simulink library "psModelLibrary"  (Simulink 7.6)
settings: Solver=ode45  SolverMode=SingleTasking  StartTime=0.0  StopTime=10.0  RelTol=1e-3
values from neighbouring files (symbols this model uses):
  psSimStruct = []    [psStartUp.m]
undefined symbols (not defined in the file or in its folder): psValve, psVolume, Restriction

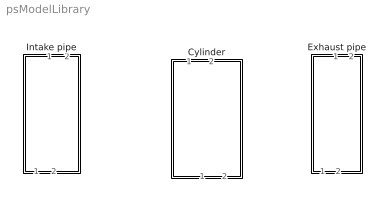
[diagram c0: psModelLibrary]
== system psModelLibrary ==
  Cylinder : Subsystem  mask{thetaOffset=0, CylNbr=1}
      mask prompts: thetaOffset "thetaOffset [rad]"; CylNbr "Cylinder Number"
  Exhaust pipe : Subsystem  mask{CylNbr=1}
      mask prompts: CylNbr "Cylinder Number"
  Intake pipe : Subsystem  mask{CylNbr=1}
      mask prompts: CylNbr "Cylinder Number"

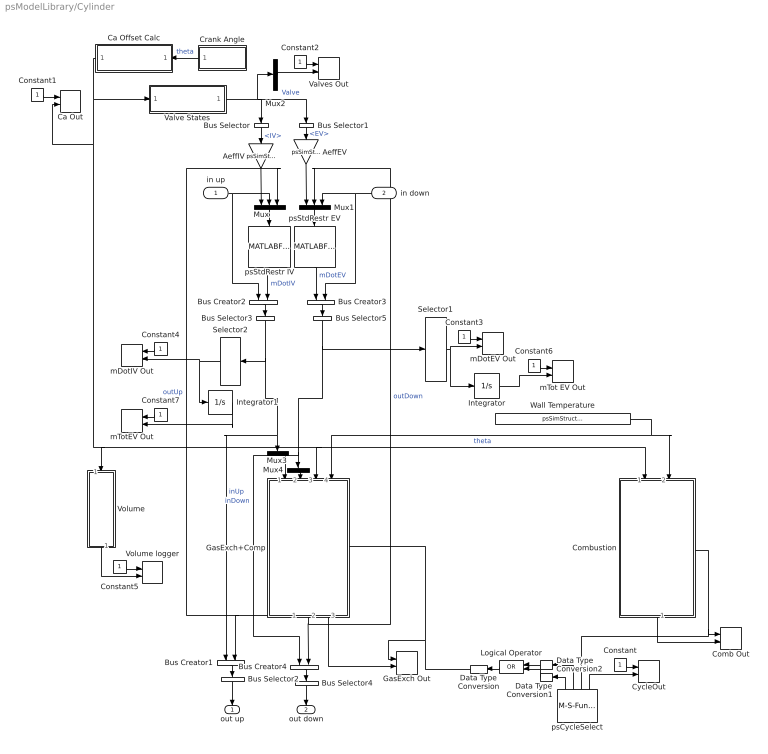
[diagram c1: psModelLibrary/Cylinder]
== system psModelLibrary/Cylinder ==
  in up : Inport
  in down : Inport  Port=2
  AeffEV : Gain  Gain=psSimStruct.psGeometry.Ath_EV*psSimStruct.psGeometry.Cd_EV
  AeffIV : Gain  Gain=psSimStruct.psGeometry.Ath_IV*psSimStruct.psGeometry.Cd_IV
  Bus Creator{1..4} (4 alike) : BusCreator  Inputs=2
  Bus Selector : BusSelector  OutputSignals=IV
  Bus Selector1 : BusSelector  OutputSignals=EV
  Bus Selector2 : BusSelector  OutputSignals=inUp.mDotIV,outUp.state  OutputAsBus=on
  Bus Selector3 : BusSelector  OutputSignals=mDotIV,signal1.state  OutputAsBus=on
  Bus Selector4 : BusSelector  OutputSignals=inDown.mDotEV,outDown.state  OutputAsBus=on
  Bus Selector5 : BusSelector  OutputSignals=mDotEV,signal2.state  OutputAsBus=on
  Ca Offset Calc : Subsystem
  Ca Out : M-S-Function  FunctionName=psToWorkspace  Parameters=1,int16('theta'),CylNbr
  Comb Out : M-S-Function  FunctionName=psToWorkspace  Parameters=9+2*psSimStruct.psThermProp.K,int16('pcb Vb Tb Vu Tu'),CylNbr
  Combustion : Subsystem  TreatAsAtomicUnit=on
  Constant{,1..7} (8 alike) : Constant
  Crank Angle : Subsystem
  CycleOut : M-S-Function  FunctionName=psToWorkspace  Parameters=1,int16('phase'),CylNbr
  Data Type Conversion : DataTypeConversion
  Data Type Conversion1 : DataTypeConversion
  Data Type Conversion2 : DataTypeConversion
  GasExch Out : M-S-Function  FunctionName=psToWorkspace  Parameters=psSimStruct.psThermProp.K+4,int16('pge Vge Tge'),CylNbr
  GasExch+Comp : Subsystem  Priority=1
  Integrator : Integrator
  Integrator1 : Integrator
  Logical Operator : Logic  Operator=OR  AllPortsSameDT=off  OutDataTypeStr=boolean
  Mux : Mux  Inputs=3
  Mux1 : Mux  Inputs=3
  Mux2 : Mux  Inputs=1
  Mux3 : Mux  Inputs=1
  Mux4 : Mux  Inputs=1
  Selector1 : Selector  IndexOptions=Index vector (dialog)  Indices=[1]  OutputSizes=[(-2)]
  Selector2 : Selector  IndexOptions=Index vector (dialog)  Indices=[1]  OutputSizes=[(-2)]
  Valve States : Subsystem
  Valves Out : M-S-Function  FunctionName=psToWorkspace  Parameters=2,int16('uIV uEV'),CylNbr
  Volume : Subsystem
  Volume logger : M-S-Function  FunctionName=psToWorkspace  Parameters=1,int16('V'),CylNbr
  Wall Temperature : Constant  Value=psSimStruct.psModel.T_Wall
  mDotEV Out : M-S-Function  FunctionName=psToWorkspace  Parameters=1,int16('mDotEV'),CylNbr
  mDotIV Out : M-S-Function  FunctionName=psToWorkspace  Parameters=1,int16('mDotIV'),CylNbr
  mTot EV Out : M-S-Function  FunctionName=psToWorkspace  Parameters=1,int16('mTotEV'),CylNbr
  mTotEV Out : M-S-Function  FunctionName=psToWorkspace  Parameters=1,int16('mTotIV'),CylNbr
  psCycleSelect : M-S-Function  FunctionName=psCycleSelect  Parameters=caOffset  mask{caOffset=thetaOffset}
      mask prompts: caOffset "caOffset [rad]"
  psStdRestr EV : MATLABFcn  MATLABFcn=psStdRestr  OutputDimensions=1  OutputSignalType=real
  psStdRestr IV : MATLABFcn  MATLABFcn=psStdRestr  OutputDimensions=1  OutputSignalType=real
  out up : Outport
  out down : Outport  Port=2
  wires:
  Constant7/1 -> mTotEV Out/1
  Integrator1/1 -> mTotEV Out/2
  Constant6/1 -> mTot EV Out/1
  Integrator/1 -> mTot EV Out/2
  Data Type Conversion2/1 -> Logical Operator/1
  Data Type Conversion1/1 -> Logical Operator/2
  Data Type Conversion/1 -> GasExch Out/1, GasExch+Comp/Enable
  Logical Operator/1 -> Data Type Conversion/1
  psCycleSelect/1 -> Data Type Conversion1/1
  psCycleSelect/2 -> Data Type Conversion2/1
  Bus Selector2/1 -> out up/1
  Bus Selector4/1 -> out down/1
  Constant4/1 -> mDotIV Out/1
  Constant3/1 -> mDotEV Out/1
  Constant2/1 -> Valves Out/1
  Constant1/1 -> Ca Out/1
  Constant/1 -> CycleOut/1
  psCycleSelect/4 -> CycleOut/2
  Combustion/1(IntOut) -> Comb Out/2
  GasExch+Comp/3(IntOut) -> GasExch Out/2
  Bus Creator4/1 -> Bus Selector4/1
  Bus Creator1/1 -> Bus Selector2/1
  psCycleSelect/3 -> Combustion/Enable, Comb Out/1
  Bus Selector5/1 -> Selector1/1, Bus Creator4/1, Mux4/1  "inDown"
  Bus Selector3/1 -> Selector2/1, Bus Creator1/1, Mux3/1  "inUp"
  Wall Temperature/1 -> GasExch+Comp/4(T_Wall), Combustion/2(Wall Temperature)
  GasExch+Comp/1(out up) -> Bus Creator1/2, Mux/3  "outUp"
  GasExch+Comp/2(out down) -> Bus Creator4/2, Mux1/2  "outDown"
  Bus Creator3/1 -> Bus Selector5/1
  Bus Creator2/1 -> Bus Selector3/1
  psStdRestr IV/1 -> Bus Creator2/2  "mDotIV"
  Crank Angle/1(theta [rad]) -> Ca Offset Calc/1(theta in)  "theta"
  Ca Offset Calc/1(theta out) -> Ca Out/2, Volume/1(theta in), Combustion/1(theta), GasExch+Comp/3(theta), Valve States/1(theta [rad])  "theta"
  Mux/1 -> psStdRestr IV/1
  Bus Selector/1 -> AeffIV/1  "<IV>"
  Mux1/1 -> psStdRestr EV/1
  Bus Selector1/1 -> AeffEV/1  "<EV>"
  psStdRestr EV/1 -> Bus Creator3/1  "mDotEV"
  in down/1 -> Bus Creator3/2, Mux1/3
  AeffIV/1 -> Mux/1
  AeffEV/1 -> Mux1/1
  Valve States/1("[iv ev]") -> Bus Selector/1, Bus Selector1/1, Mux2/1  "Valve"
  in up/1 -> Bus Creator2/1, Mux/2
  Selector1/1 -> Integrator/1, mDotEV Out/2
  Selector2/1 -> Integrator1/1, mDotIV Out/2
  Constant5/1 -> Volume logger/1
  Volume/1(V) -> Volume logger/2
  Mux2/1 -> Valves Out/2
  Mux3/1 -> GasExch+Comp/1(inUp)
  Mux4/1 -> GasExch+Comp/2(inDown)

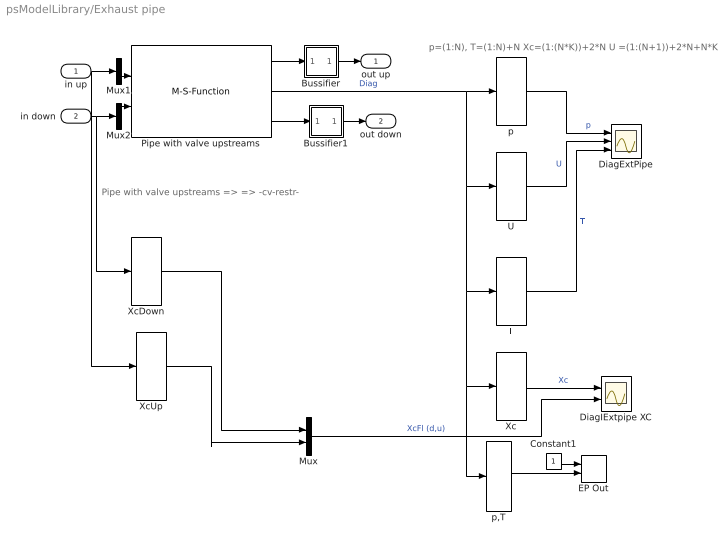
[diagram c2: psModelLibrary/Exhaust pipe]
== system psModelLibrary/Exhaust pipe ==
  note: p=(1:N), T=(1:N)+N Xc=(1:(N*K))+2*N U =(1:(N+1))+2*N+N*K
  note: Pipe with valve upstreams => => -cv-restr-
  in up : Inport
  in down : Inport  Port=2
  Bussifier : Subsystem
  Bussifier1 : Subsystem
  Constant1 : Constant
  DiagExtPipe : Scope  NumInputPorts=3
  DiagIExtpipe XC : Scope  NumInputPorts=2
  EP Out : M-S-Function  FunctionName=psToWorkspace  Parameters=4,int16('pEP_U pEP_D TEP_U TEP_D'),CylNbr
  Mux : Mux  Inputs=2
  Mux1 : Mux  Inputs=1
  Mux2 : Mux  Inputs=1
  Pipe with valve upstreams : M-S-Function  FunctionName=psMultiGasPipe  Parameters=N,NumInputs,x,A,Pinit,Tinit,propInit,kFric,connectorUp,connectorDown  mask{N=psSimStruct.psModel.N_pipe, NumInputs=[1,1], x=psSimStruct.psModel.length_pipe_EM, A=psSimStruct.psModel.area_pipe_EM, Pinit=psSimStruct.psModel.pIC_EM, Tinit=psSimStruct.psModel.TIC_EM, propInit=psSimStruct.psModel.XgcIC_EM, kFric=psSimStruct.psModel.friction_EM, connectorUp=Restriction, connectorDown=Control Volume}
      mask prompts: N "Number of elements"; NumInputs "Number of Inputs"; x "Pipe length [m]"; A "Pipe Area [m2]"; Pinit "Initial Pressure [Pa]"; Tinit "Initial Temperature [K]"; propInit "Initial prop [-]"; kFric "Pipe Friction"; connectorUp "Upstreams connector"; connectorDown "Downstreams connector"
  T : Selector  IndexOptions=Index vector (dialog)  Indices=(1:psSimStruct.psModel.N_pipe)+psSimStruct.psModel.N_pipe  OutputSizes=[(-2)]
  U : Selector  IndexOptions=Index vector (dialog)  Indices=(1:(psSimStruct.psModel.N_pipe+1))+2*psSimStruct.psModel.N_pipe+psSimStruct.psModel.N_pipe*psSimStruct.psThermProp.K  OutputSizes=[(-2)]
  Xc : Selector  IndexOptions=Index vector (dialog)  Indices=2*psSimStruct.psModel.N_pipe+1:(psSimStruct.psModel.N_pipe*psSimStruct.psThermProp.K)  OutputSizes=[(-2)]
  XcDown : Selector  IndexOptions=Index vector (dialog)  Indices=[3+(1:psSimStruct.psThermProp.K)]  OutputSizes=1
  XcUp : Selector  IndexOptions=Index vector (dialog)  Indices=3+(1:psSimStruct.psThermProp.K)  OutputSizes=1
  p : Selector  IndexOptions=Index vector (dialog)  Indices=1:psSimStruct.psModel.N_pipe  OutputSizes=[(-2)]
  p,T : Selector  IndexOptions=Index vector (dialog)  Indices="[1 psSimStruct.psModel.N_pipe psSimStruct.psModel.N_pipe+1  psSimStruct.psModel.N_pipe*2]"  OutputSizes=[(-2)]
  out up : Outport
  out down : Outport  Port=2
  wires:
  Mux/1 -> DiagIExtpipe XC/2  "XcFl (d,u)"
  Constant1/1 -> EP Out/1
  p,T/1 -> EP Out/2
  Xc/1 -> DiagIExtpipe XC/1  "Xc"
  T/1 -> DiagExtPipe/3  "T"
  p/1 -> DiagExtPipe/1  "p"
  Pipe with valve upstreams/2 -> p,T/1, Xc/1, T/1, U/1, p/1  "Diag"
  U/1 -> DiagExtPipe/2  "U"
  Pipe with valve upstreams/1 -> Bussifier/1(In1)
  in down/1 -> XcDown/1, Mux2/1
  in up/1 -> XcUp/1, Mux1/1
  Pipe with valve upstreams/3 -> Bussifier1/1(In1)
  XcDown/1 -> Mux/1
  XcUp/1 -> Mux/2
  Bussifier1/1(Out1) -> out down/1
  Bussifier/1(Out1) -> out up/1
  Mux1/1 -> Pipe with valve upstreams/1
  Mux2/1 -> Pipe with valve upstreams/2

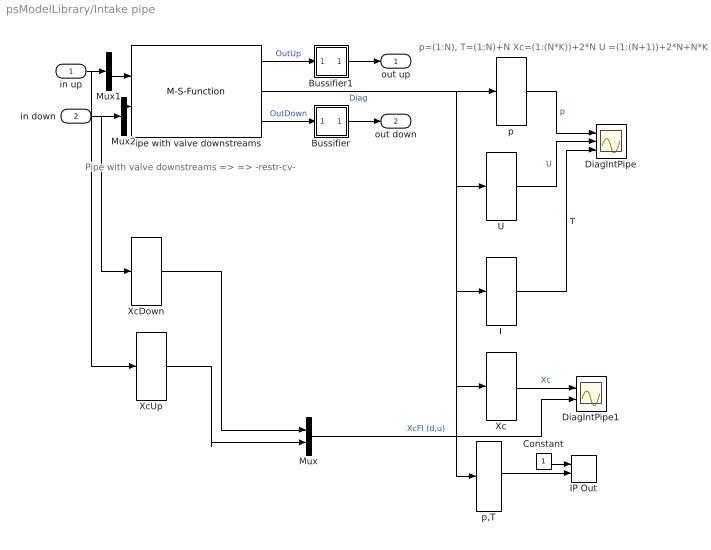
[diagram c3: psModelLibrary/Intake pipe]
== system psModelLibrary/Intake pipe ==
  note: p=(1:N), T=(1:N)+N Xc=(1:(N*K))+2*N U =(1:(N+1))+2*N+N*K
  note: Pipe with valve downstreams => => -restr-cv-
  in up : Inport
  in down : Inport  Port=2
  Bussifier : Subsystem
  Bussifier1 : Subsystem
  Constant : Constant
  DiagIntPipe : Scope  NumInputPorts=3
  DiagIntPipe1 : Scope  NumInputPorts=2
  IP Out : M-S-Function  FunctionName=psToWorkspace  Parameters=4,int16('pIP_U pIP_D TIP_U TIP_D'),CylNbr
  Mux : Mux  Inputs=2
  Mux1 : Mux  Inputs=1
  Mux2 : Mux  Inputs=1
  Pipe with valve downstreams : M-S-Function  FunctionName=psMultiGasPipe  Parameters=N,NumInputs,x,A,Pinit,Tinit,propInit,kFric,connectorUp,connectorDown  mask{N=psSimStruct.psModel.N_pipe, NumInputs=[1,1], x=psSimStruct.psModel.length_pipe_IM, A=psSimStruct.psModel.area_pipe_IM, Pinit=psSimStruct.psModel.pIC_IM, Tinit=psSimStruct.psModel.TIC_IM, propInit=psSimStruct.psModel.XgcIC_IM, kFric=psSimStruct.psModel.friction_IM, connectorUp=Control Volume, connectorDown=Restriction}
      mask prompts: N "Number of elements"; NumInputs "Number of Inputs"; x "Pipe length [m]"; A "Pipe Area [m2]"; Pinit "Initial Pressure [Pa]"; Tinit "Initial Temperature [K]"; propInit "Initial prop [-]"; kFric "Pipe Friction"; connectorUp "Upstreams connector"; connectorDown "Downstreams connector"
  T : Selector  IndexOptions=Index vector (dialog)  Indices=(1:psSimStruct.psModel.N_pipe)+psSimStruct.psModel.N_pipe  OutputSizes=[(-2)]
  U : Selector  IndexOptions=Index vector (dialog)  Indices=(1:(psSimStruct.psModel.N_pipe+1))+2*psSimStruct.psModel.N_pipe+psSimStruct.psModel.N_pipe*psSimStruct.psThermProp.K  OutputSizes=[(-2)]
  Xc : Selector  IndexOptions=Index vector (dialog)  Indices=2*psSimStruct.psModel.N_pipe+(1:(psSimStruct.psModel.N_pipe*psSimStruct.psThermProp.K))  OutputSizes=[(-2)]
  XcDown : Selector  IndexOptions=Index vector (dialog)  Indices=[3+(1:psSimStruct.psThermProp.K)]  OutputSizes=1
  XcUp : Selector  IndexOptions=Index vector (dialog)  Indices=3+(1:psSimStruct.psThermProp.K)  OutputSizes=1
  p : Selector  IndexOptions=Index vector (dialog)  Indices=1:psSimStruct.psModel.N_pipe  OutputSizes=[(-2)]
  p,T : Selector  IndexOptions=Index vector (dialog)  Indices="[1 psSimStruct.psModel.N_pipe psSimStruct.psModel.N_pipe+1  psSimStruct.psModel.N_pipe*2]"  OutputSizes=[(-2)]
  out up : Outport
  out down : Outport  Port=2
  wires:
  Mux/1 -> DiagIntPipe1/2  "XcFl (d,u)"
  XcDown/1 -> Mux/1
  XcUp/1 -> Mux/2
  Constant/1 -> IP Out/1
  p,T/1 -> IP Out/2
  Xc/1 -> DiagIntPipe1/1  "Xc"
  T/1 -> DiagIntPipe/3  "T"
  in up/1 -> XcUp/1, Mux1/1
  in down/1 -> XcDown/1, Mux2/1
  Pipe with valve downstreams/1 -> Bussifier1/1(In1)  "OutUp"
  Bussifier/1(Out1) -> out down/1
  Bussifier1/1(Out1) -> out up/1
  p/1 -> DiagIntPipe/1  "p"
  Pipe with valve downstreams/3 -> Bussifier/1(In1)  "OutDown"
  Pipe with valve downstreams/2 -> p,T/1, Xc/1, T/1, U/1, p/1  "Diag"
  U/1 -> DiagIntPipe/2  "U"
  Mux1/1 -> Pipe with valve downstreams/1
  Mux2/1 -> Pipe with valve downstreams/2

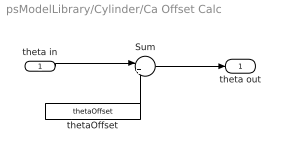
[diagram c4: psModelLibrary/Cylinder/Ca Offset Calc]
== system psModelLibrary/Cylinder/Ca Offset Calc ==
  theta in : Inport
  Sum : Sum  Inputs=|++
  thetaOffset : Constant  Value=thetaOffset
  theta out : Outport
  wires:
  thetaOffset/1 -> Sum/2
  theta in/1 -> Sum/1
  Sum/1 -> theta out/1

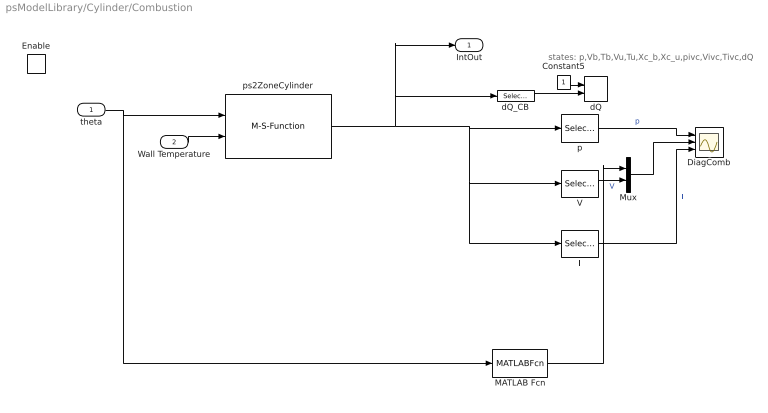
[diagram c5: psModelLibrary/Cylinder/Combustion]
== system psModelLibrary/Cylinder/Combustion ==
  note: states: p,Vb,Tb,Vu,Tu,Xc_b,Xc_u,pivc,Vivc,Tivc,dQ
  theta : Inport
  Wall Temperature : Inport  Port=2
  Enable : EnablePort  StatesWhenEnabling=reset
  Constant5 : Constant
  DiagComb : Scope  NumInputPorts=3
  MATLAB Fcn : MATLABFcn  MATLABFcn=psVolume(u(1))  OutputDimensions=1
  Mux : Mux  Inputs=2
  T : Selector  IndexOptions=Index vector (dialog)  Indices=[3 5]  OutputSizes=[(-2)]
  V : Selector  IndexOptions=Index vector (dialog)  Indices=[2 4]  OutputSizes=[(-2)]
  dQ : M-S-Function  FunctionName=psToWorkspace  Parameters=1,int16('dQ'),CylNbr
  dQ_CB : Selector  IndexOptions=Index vector (dialog)  Indices=[psSimStruct.psThermProp.K*2+9]  OutputSizes=[(-2)]
  p : Selector  IndexOptions=Index vector (dialog)  Indices=[1]  OutputSizes=[(-2)]
  ps2ZoneCylinder : M-S-Function  FunctionName=ps2ZoneCylinder  Parameters=thetaOffset,CylNbr
  IntOut : Outport
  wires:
  Wall Temperature/1 -> ps2ZoneCylinder/2
  theta/1 -> ps2ZoneCylinder/1, MATLAB Fcn/1
  MATLAB Fcn/1 -> Mux/1
  Mux/1 -> DiagComb/2
  V/1 -> Mux/2  "V"
  T/1 -> DiagComb/3  "T"
  p/1 -> DiagComb/1  "p"
  ps2ZoneCylinder/1 -> T/1, V/1, p/1, IntOut/1, dQ_CB/1
  Constant5/1 -> dQ/1
  dQ_CB/1 -> dQ/2

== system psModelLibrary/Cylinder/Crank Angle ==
  simulation time : Clock
  speed : Gain  Gain=psSimStruct.psSimPar.w
  theta [rad] : Outport
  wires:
  simulation time/1 -> speed/1
  speed/1 -> theta [rad]/1

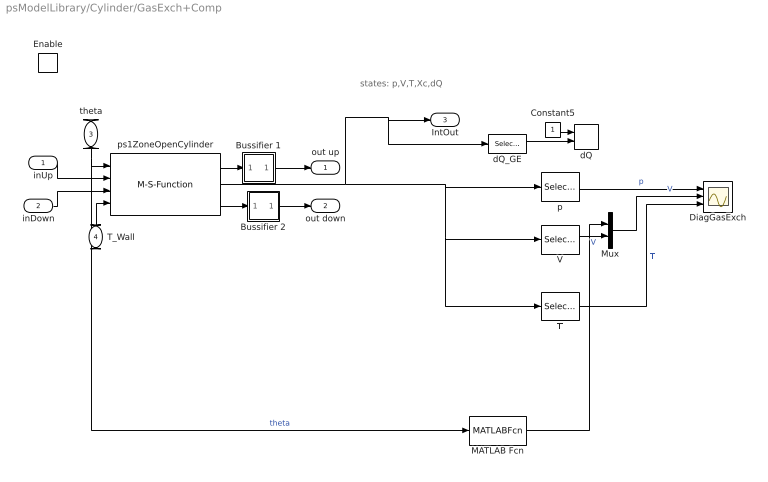
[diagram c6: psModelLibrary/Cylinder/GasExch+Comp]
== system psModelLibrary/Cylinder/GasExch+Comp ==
  note: states: p,V,T,Xc,dQ
  inUp : Inport
  inDown : Inport  Port=2
  theta : Inport  Port=3
  T_Wall : Inport  Port=4
  Enable : EnablePort  StatesWhenEnabling=reset
  Bussifier 1 : Subsystem
  Bussifier 2 : Subsystem
  Constant5 : Constant
  DiagGasExch : Scope  NumInputPorts=3
  MATLAB Fcn : MATLABFcn  MATLABFcn=psVolume(u(1))  OutputDimensions=1
  Mux : Mux  Inputs=2
  T : Selector  IndexOptions=Index vector (dialog)  Indices=[3]  OutputSizes=[(-2)]
  V : Selector  IndexOptions=Index vector (dialog)  Indices=[2]  OutputSizes=[(-2)]
  dQ : M-S-Function  FunctionName=psToWorkspace  Parameters=1,int16('dQ'),CylNbr
  dQ_GE : Selector  IndexOptions=Index vector (dialog)  Indices=[psSimStruct.psThermProp.K+4]  OutputSizes=[(-2)]
  p : Selector  IndexOptions=Index vector (dialog)  Indices=[1]  OutputSizes=[(-2)]
  ps1ZoneOpenCylinder : M-S-Function  FunctionName=ps1ZoneOpenCylinder  Parameters=thetaOffset,CylNbr
  out up : Outport  InitialOutput=[0 1e5 300 psSimStruct.psModel.XgcAmb]
  out down : Outport  Port=2  InitialOutput=[0 1e5 300 psSimStruct.psModel.XgcAmb]
  IntOut : Outport  Port=3
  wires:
  MATLAB Fcn/1 -> Mux/1
  Mux/1 -> DiagGasExch/2  "V"
  V/1 -> Mux/2  "V"
  T/1 -> DiagGasExch/3  "T"
  p/1 -> DiagGasExch/1  "p"
  ps1ZoneOpenCylinder/2 -> V/1, T/1, p/1, IntOut/1, dQ_GE/1
  ps1ZoneOpenCylinder/3 -> Bussifier 2/1(In1)
  ps1ZoneOpenCylinder/1 -> Bussifier 1/1(In1)
  inDown/1 -> ps1ZoneOpenCylinder/3
  inUp/1 -> ps1ZoneOpenCylinder/2
  theta/1 -> MATLAB Fcn/1, ps1ZoneOpenCylinder/1  "theta"
  T_Wall/1 -> ps1ZoneOpenCylinder/4
  Bussifier 2/1(Out1) -> out down/1
  Bussifier 1/1(Out1) -> out up/1
  Constant5/1 -> dQ/1
  dQ_GE/1 -> dQ/2

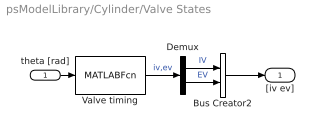
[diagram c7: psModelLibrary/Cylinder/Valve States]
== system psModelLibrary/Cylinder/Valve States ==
  theta [rad] : Inport
  Bus Creator2 : BusCreator  Inputs=2
  Demux : Demux  Outputs=2
  Valve timing : MATLABFcn  Description=|  MATLABFcn=psValve(u(1))  OutputDimensions=2
      | [u] = psValve(CA)                                   
      | Calculates the valve states. u = [u1 u2]', where u1  
      | is the intake valve and u2 the outlet valve.         
      | u1, u2 = 1 means fully open, u1, u2 = 0 means closed.
  "[iv ev]" : Outport
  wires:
  theta [rad]/1 -> Valve timing/1
  Demux/1 -> Bus Creator2/1  "IV"
  Demux/2 -> Bus Creator2/2  "EV"
  Bus Creator2/1 -> "[iv ev]"/1
  Valve timing/1 -> Demux/1  "iv,ev"

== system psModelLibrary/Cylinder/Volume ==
  theta in : Inport
  Total Volume : MATLABFcn  Description=|  MATLABFcn=psVolume(u(1))  OutputDimensions=1
      | [u] = psValve(CA)                                   
      | Calculates the valve states. u = [u1 u2]', where u1  
      | is the intake valve and u2 the outlet valve.         
      | u1, u2 = 1 means fully open, u1, u2 = 0 means closed.
  V : Outport
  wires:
  theta in/1 -> Total Volume/1
  Total Volume/1 -> V/1

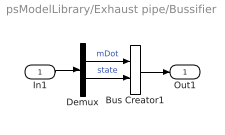
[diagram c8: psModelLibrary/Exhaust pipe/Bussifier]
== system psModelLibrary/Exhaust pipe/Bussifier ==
  In1 : Inport
  Bus Creator1 : BusCreator  Inputs=2
  Demux : Demux  Outputs=[1 2+psSimStruct.psThermProp.K]
  Out1 : Outport
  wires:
  In1/1 -> Demux/1
  Bus Creator1/1 -> Out1/1
  Demux/2 -> Bus Creator1/2  "state"
  Demux/1 -> Bus Creator1/1  "mDot"

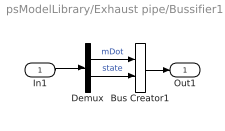
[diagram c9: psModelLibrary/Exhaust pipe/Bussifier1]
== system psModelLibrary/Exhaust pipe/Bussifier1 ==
  In1 : Inport
  Bus Creator1 : BusCreator  Inputs=2
  Demux : Demux  Outputs=[1 2+psSimStruct.psThermProp.K]
  Out1 : Outport
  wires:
  Demux/1 -> Bus Creator1/1  "mDot"
  Demux/2 -> Bus Creator1/2  "state"
  Bus Creator1/1 -> Out1/1
  In1/1 -> Demux/1

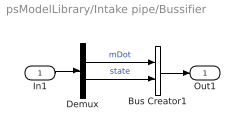
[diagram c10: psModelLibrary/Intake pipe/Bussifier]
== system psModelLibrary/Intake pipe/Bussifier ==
  In1 : Inport
  Bus Creator1 : BusCreator  Inputs=2
  Demux : Demux  Outputs=[1 2+psSimStruct.psThermProp.K]
  Out1 : Outport
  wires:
  Demux/1 -> Bus Creator1/1  "mDot"
  Demux/2 -> Bus Creator1/2  "state"
  Bus Creator1/1 -> Out1/1
  In1/1 -> Demux/1

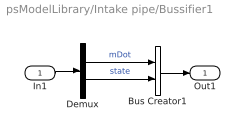
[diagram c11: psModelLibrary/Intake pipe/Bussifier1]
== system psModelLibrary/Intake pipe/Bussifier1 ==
  In1 : Inport
  Bus Creator1 : BusCreator  Inputs=2
  Demux : Demux  Outputs=[1 2+psSimStruct.psThermProp.K]
  Out1 : Outport
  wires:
  In1/1 -> Demux/1
  Bus Creator1/1 -> Out1/1
  Demux/2 -> Bus Creator1/2  "state"
  Demux/1 -> Bus Creator1/1  "mDot"

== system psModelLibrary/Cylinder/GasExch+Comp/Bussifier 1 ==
  In1 : Inport
  Bus Creator2 : BusCreator  Inputs=2
  Ground : Ground
  Out1 : Outport
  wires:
  Ground/1 -> Bus Creator2/1  "mDot"
  In1/1 -> Bus Creator2/2  "state"
  Bus Creator2/1 -> Out1/1

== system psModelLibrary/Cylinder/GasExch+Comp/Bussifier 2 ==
  In1 : Inport
  Bus Creator2 : BusCreator  Inputs=2
  Ground : Ground
  Out1 : Outport
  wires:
  Bus Creator2/1 -> Out1/1
  In1/1 -> Bus Creator2/2  "state"
  Ground/1 -> Bus Creator2/1  "mDot"
